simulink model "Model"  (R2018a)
settings: Solver=ode15s  StartTime=0.0  StopTime=tsim  RelTol=1e-5
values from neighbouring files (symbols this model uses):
  C = Fc*cpc/(Fh*cph)    [calcblock.m]    (also in eNTU.m = m.c*cp.c/(m.h*cp.h); Main.m = [zeros(1,2*N-1),1]; Main_OL.m = [zeros(1,2*N-1),1]; testfun.m = mc*cpc/(mh*cph))
  d0 = [Fh, Tcin, Thin]    [Main.m]    (also in Main_OL.m; runTestCalcBlk.m; runTransf.m = [Fh; Tcin; U0; Ffeed0; m0; Tfeed0]; runTransfOL.m)
  d_step = [Fh, Tcin, Thin]    [Main.m]    (also in Main_OL.m = [Fh, Tcin+0, Thin]; runTestCalcBlk.m)
  d_tstep = [1000; 1000;2000]    [Main.m]    (also in Main_OL.m = 300; runTestCalcBlk.m = 300; runTransf.m = [500; 50000; 70000; 130000; 50000; 50000]; runTransfOL.m = [500 5000 7000 13000])
  Fc0 = 5    [Main.m]    (also in Main_OL.m; runTestCalcBlk.m; runTransf.m; runTransfOL.m)
  KI = Kp/tauIv    [Main.m]    (also in Main_OL.m = 1; runTransf.m = 1/kS(i)*1/tauCS(i); runTransfOL.m = 1/kS(i)*1/tauCS(i))
  nd = size(d0,2)    [Main.m]    (also in Main_OL.m; runTestCalcBlk.m; runTransf.m = size(d0,1); runTransfOL.m)
  np = size(p,2)    [Main.m]    (also in Main_OL.m; runH2Psim.m = length(param); runTestCalcBlk.m; runTransf.m)
  nu = 1    [Main.m]    (also in Main_OL.m; runH2Psim.m = length(u0); runTestCalcBlk.m; runTransf.m)
  nx = size(x0,1)    [Main.m]    (also in Main_OL.m; H2P_Turbine_driven.m = param(end); runTD.m = length(x0); H2P_Boiler_driven.m = param(end))
  p = [N, Fc0, rhoc, rhoh,U,A,cpc,cph]    [Main.m]    (also in Main_OL.m; runTestCalcBlk.m; NonlinearMap.m = [U;A;Fc(i);Fh;cpc;cph;Tcin;Thin]; runTransf.m = [N, Fc0, rhoc, rhoh, U0, A,cpc,cph])
  Thsp = Thsp0+dThsp    [Main.m]    (also in Main_OL.m; runTestCalcBlk.m; runTransf.m = Thsp0; runTransfOL.m = Thsp0)
  Thsp0 = Thend(end)    [Main.m]    (also in Main_OL.m = 297.120261168; runTestCalcBlk.m; runTransf.m = x0(end-1);  2.971202611676064e+02; runTransfOL.m = x0(end);  2.971202611676064e+02)
  tstep = 100    [Main_OL.m]    (also in Main.m; runTransf.m = 10000; runTransfOL.m)
  v0 = Tout.h    [Main.m]    (also in Main_OL.m = 1; runTD.m = v(end,:); runBD.m = v(end,:); runFP.m = v(end,:))
  x0 = [Tcend(1:N)'; Thend(1:N)']    [Main.m]    (also in Main_OL.m; runTD.m = [TE0;TD0;TSh0;MD0; MSh0;w0;TA0;0;0;0;0;0;0;0;0;0]; runBD.m = [TE0;TD0;TSh0;MD0; MSh0;w0;TA0;0;0;0;0;0;0;0;0;0]; runFP.m = [TE0;TD0;TSh0;MD0; MSh0;w0;TA0;0;0;0;0;0;0;0])
undefined symbols (not defined in the file or in its folder): calcblock, HEXode

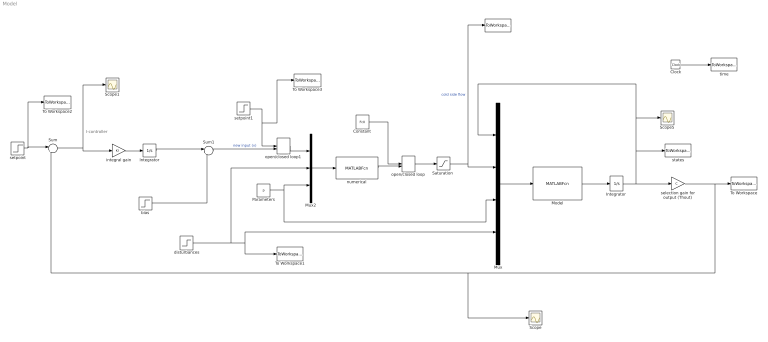
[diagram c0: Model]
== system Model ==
  note: I-controller
  " " : ToWorkspace  VariableName=uc  SampleTime=-1
  Clock : Clock
  Constant : Constant  Value=Fc0
  Integrator : Integrator
  "Integrator " : Integrator  InitialCondition=x0
  Model : MATLABFcn  MATLABFcn=HEXode(u(1:nx),u(nx+1:nx+nu),u(nx+nu+1:nx+nu+np),u(nx+nu+np+1:nx+nu+np+nd))  OutputDimensions=nx  Output1D=off
  Mux : Mux
  Mux2 : Mux  Inputs=3
  Parameters : Constant  Value=p
  "Saturation " : Saturate  UpperLimit=inf  LowerLimit=0
  Scope : Scope
  Scope1 : Scope
  Scope5 : Scope
  Sum : Sum  Inputs=|+-
  Sum1 : Sum  Inputs=|++
  To Workspace : ToWorkspace  VariableName=Thout  SampleTime=-1
  To Workspace1 : ToWorkspace  VariableName=dsim  SampleTime=-1
  To Workspace2 : ToWorkspace  VariableName=Tsp  SampleTime=-1
  To Workspace3 : ToWorkspace  VariableName=ysp  SampleTime=-1
  bias : Step  Time=d_tstep  Before=v0  After=v0  SampleTime=0
  disturbances : Step  Time=d_tstep  Before=d0  After=d_step  SampleTime=0
  integral gain : Gain  Gain=KI  Multiplication=Matrix(K*u)
  numerical : MATLABFcn  MATLABFcn=calcblock(u(nu),u(nu+1:nu+nd),u(nu+nd+1:nu+nd+np))
  open/closed loop : ManualSwitch  CurrentSetting=0
  open/closed loop1 : ManualSwitch
  selection gain for output (Thout) : Gain  Gain=C  Multiplication=Matrix(K*u)
  setpoint : Step  Before=Thsp0  After=Thsp  SampleTime=0
  setpoint1 : Step  Time=tstep  Before=Thsp0  After=Thsp  SampleTime=0
  states : ToWorkspace  VariableName=T  SampleTime=-1
  time : ToWorkspace  VariableName=t  SampleTime=-1
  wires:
  Model/1 -> "Integrator "/1
  "Integrator "/1 -> states/1, Mux/1, Scope5/1, selection gain for output (Thout)/1
  Mux/1 -> Model/1
  Clock/1 -> time/1
  Parameters/1 -> Mux/3, Mux2/3
  disturbances/1 -> Mux2/2, To Workspace1/1, Mux/4
  "Saturation "/1 -> " "/1, Mux/2  "cold side flow"
  numerical/1 -> open/closed loop/2
  setpoint/1 -> To Workspace2/1, Sum/1
  Sum/1 -> Scope1/1, integral gain/1
  integral gain/1 -> Integrator/1
  Sum1/1 -> open/closed loop1/2  "new input (v)"
  selection gain for output (Thout)/1 -> Sum/2, Scope/1, To Workspace/1
  Mux2/1 -> numerical/1
  bias/1 -> Sum1/2
  open/closed loop/1 -> "Saturation "/1
  Constant/1 -> open/closed loop/1
  Integrator/1 -> Sum1/1
  open/closed loop1/1 -> Mux2/1
  setpoint1/1 -> To Workspace3/1, open/closed loop1/1
